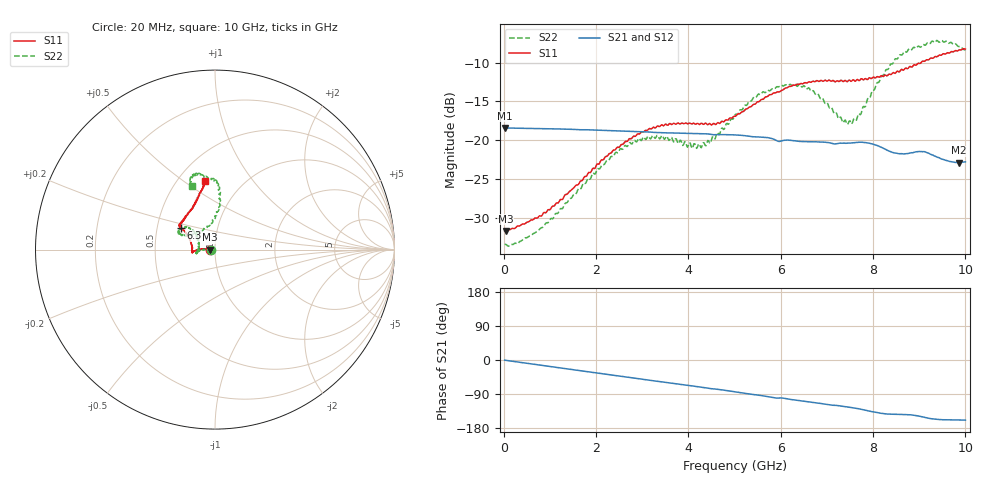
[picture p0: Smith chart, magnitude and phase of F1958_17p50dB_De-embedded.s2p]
! Integrated Device Technology
! Corporate Headquarters
! 6024 Silver Creek Valley Road
! San Jose, CA 95138  USA
! Phone:  1-408-284-8200
! Toll Free:  1-800-223-1366
! Webpage:  http://www.idt.com/
! Timing and RF Division
! 515 Groton Road, Suite 102
! Westford, MA 01886-6024
! Device:  F1958
! Description: 7-bit 0.25 dB Digital Step Attenuator
! Frequency:  0.001 -  6.000 GHz
! Package:  4x4 mm Thin QFN Plastic Package: 24 pin
! Ports:  2 RF, 12 DC
!  Pin  1  = D0
!  Pin  2  = VDD
!  Pin  3  = VMODE
!  Pin  4  = GND
!  Pin  5  = RF1  =  Port 1
!  Pin  6  = GND
!  Pin  7  = GND
!  Pin  8  = GND
!  Pin  9  = GND
!  Pin 10  = GND
!  Pin 11  = GND
!  Pin 12  = GND
!  Pin 13  = GND
!  Pin 14  = RF2  =  Port 2
!  Pin 15  = GND
!  Pin 16  = LE
!  Pin 17  = CLK
!  Pin 18  = DATA
!  Pin 19  = D6
!  Pin 20  = D5
!  Pin 21  = D4
!  Pin 22  = D3
!  Pin 23  = D2
!  Pin 24  = D1
! State:  70
! Atten State:  17.50 dB
! Voltage:  +3.30 Volts
! Current:  0.258 mA
! Data:  The device was measured on a F1958 evaluation board which has
!  individual transmission lines to the RF pins.  Data was collected
!  using a calibrated network analyzer.  The evaluation board was
!  de-embedded using Automatic Fixture Removal (AFR).
!  The reference plane is the edge of the package pin.
! Misc:
!  Action Tracker AT0419
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# GHz S dB R 50
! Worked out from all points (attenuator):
!   500 points, 20 MHz to 10 GHz, reference 50 ohm
!   highest |S21| = -18.39 dB at 20 MHz (marker M1); lowest = -22.9 dB at 9.86 GHz (marker M2)
!   lowest |S11| = -31.6 dB at 40 MHz (marker M3), VSWR 1.05, Z = 47.4 - j0.0715 ohm
!   |S11| at or under -10 dB: start of sweep to 9.042 GHz
!   |S22| runs from -33.6 to -7.2 dB; largest |S21 - S12| = 0.0004
!   S11 on the Smith chart (normalised r, x): 20 MHz: 0.95, -0.00; 6.3 GHz: 0.66, +0.17; 10 GHz: 0.67, +0.60
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0.02  -31.60 -178.3  -18.39 -0.5  -18.39 -0.4  -33.37 -178.2
0.04  -31.63 -178.4  -18.40 -0.8  -18.39 -0.8  -33.33 -177.4
0.3  -30.99 176.9  -18.43 -5.3  -18.43 -5.3  -33.27 178.4
0.72  -29.99 176.4  -18.48 -12.4  -18.47 -12.4  -31.69 178.1
1.7  -25.16 176.2  -18.63 -28.9  -18.62 -28.9  -25.81 178.0
2.62  -20.22 -179.2  -18.82 -44.3  -18.80 -44.3  -20.67 -175.6
2.92  -19.17 -176.2  -18.87 -49.3  -18.86 -49.4  -19.76 -172.8
3.36  -18.21 -173.4  -19.00 -56.7  -19.00 -56.8  -19.64 -167.9
4.3  -17.83 -178.6  -19.14 -72.1  -19.15 -72.1  -20.64 164.1
4.64  -17.71 172.9  -19.27 -77.5  -19.28 -77.5  -19.03 151.6
5.02  -16.90 161.8  -19.30 -84.1  -19.31 -84.1  -16.65 140.5
5.56  -14.86 151.0  -19.57 -93.6  -19.58 -93.5  -14.13 141.4
6.3  -12.92 147.9  -20.05 -105.5  -20.06 -105.5  -12.75 153.4
6.68  -12.45 146.0  -20.18 -111.3  -20.19 -111.3  -13.67 155.5
7.32  -12.30 140.2  -20.37 -121.8  -20.37 -121.7  -17.31 135.7
7.5  -12.30 137.1  -20.35 -124.7  -20.35 -124.6  -17.49 118.0
7.7  -12.34 133.1  -20.23 -128.9  -20.24 -128.9  -16.57 101.0
8.34  -11.51 118.1  -21.35 -142.8  -21.36 -143.0  -10.74 84.1
8.68  -10.86 111.5  -21.73 -143.9  -21.72 -143.9  -8.56 88.2
9.26  -9.42 103.5  -21.82 -154.8  -21.83 -154.9  -7.38 100.6
9.86  -8.41 98.6  -22.85 -158.1  -22.89 -157.9  -7.96 109.3
10  -8.27 98.5  -22.76 -158.6  -22.77 -158.5  -8.43 110.1
